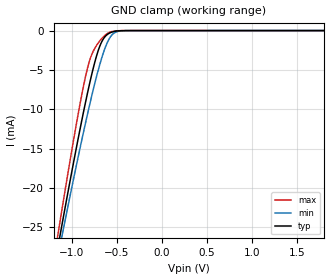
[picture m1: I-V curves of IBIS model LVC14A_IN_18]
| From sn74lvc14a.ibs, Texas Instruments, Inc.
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[Model]   LVC14A_IN_18
Model_type  Input
Vinh=0.85
Vinl=0.4
| variable   typ   min   max
C_comp   2.63pF   2.15pF   3.13pF
[Temperature Range]   40   100   -40
| Ambient temperature   25   85   -40
[Voltage range]   1.8   1.65   1.95
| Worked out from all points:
|   GND clamp passes 1 mA (typ) near -0.64 V on its own axis
[GND Clamp]
| LVC14A_IN_18
|   Voltage   I(typ)   I(min)   I(max)
-5.5V     -338.9mA   -314.3mA   -369mA
-1.16V    -28.09mA   -29.24mA   -26.56mA
-1.12V    -25.56mA   -26.92mA   -23.71mA
-1.085V   -23.36mA   -24.91mA   -21.25mA
-925mV    -13.65mA   -15.98mA   -10.52mA
-820mV    -7.797mA   -10.48mA   -4.654mA
-770mV    -5.293mA   -8.026mA   -2.891mA
-695mV    -2.253mA   -4.666mA   -1.432mA
-600mV    -473.7uA   -1.449mA   -358.4uA
-535mV    -136.2uA   -379.8uA   -78.5uA
-445mV    -16.2uA    -36.49uA   -4.833uA
1.8V      41.95pA    147.4pA    23.47pA
